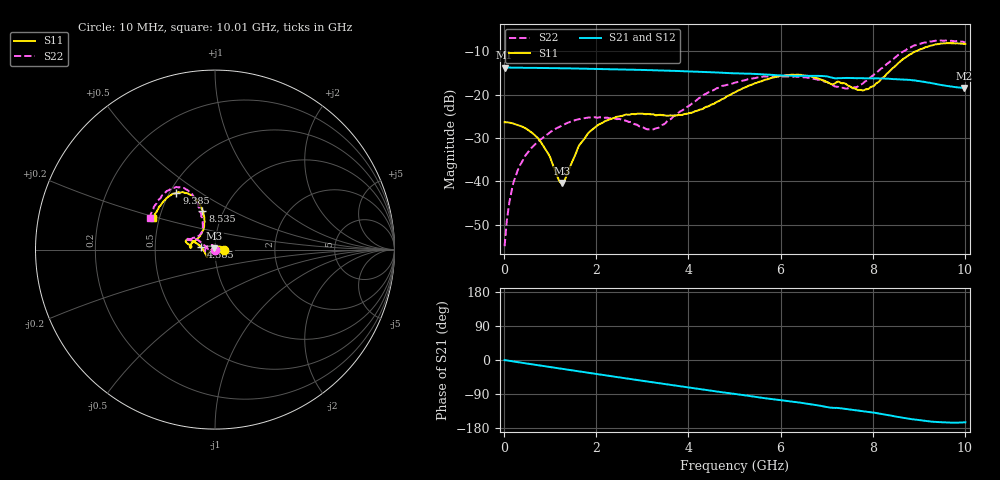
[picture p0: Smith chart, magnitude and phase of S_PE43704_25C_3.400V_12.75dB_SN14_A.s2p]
! Device ID: PE43704
! Dir: z:\PE43704\PE43704_Char_1_20130516\PE43704\AMB\3p400V\12p75dB
! Serial: 14
! Insertion: A
! Impedance: 50 ohm
! Temp: Amb
! VDD: 3.400V
! Attenuation Step: 12.75dB
! IDD: 1.140121e-01mA
#  Hz  S  RI  R  50
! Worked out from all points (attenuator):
!   401 points, 10 MHz to 10.01 GHz, reference 50 ohm
!   highest |S21| = -13.73 dB at 10 MHz (marker M1); lowest = -18.4 dB at 9.985 GHz (marker M2)
!   lowest |S11| = -40.4 dB at 1.26 GHz (marker M3), VSWR 1.02, Z = 49.5 + j0.822 ohm
!   |S11| at or under -10 dB: start of sweep to 8.933 GHz
!   |S22| runs from -54.9 to -7.5 dB; largest |S21 - S12| = 0.0015
!   S11 on the Smith chart (normalised r, x): 10 MHz: 1.10, +0.00; 4.585 GHz: 0.85, +0.03; 8.535 GHz: 0.80, +0.36; 9.385 GHz: 0.54, +0.40; 10.01 GHz: 0.46, +0.19
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1e7  0.0482 0.000196  0.2059 -0.000751  0.2061 -0.000737  0.00174 0.000404
1.6e8  0.0469 0.00473  0.2051 -0.0113  0.2052 -0.0111  0.00161 0.00748
3.6e8  0.0422 0.0106  0.2037 -0.0245  0.2035 -0.0247  -0.00204 0.0158
7.85e8  0.0233 0.0174  0.1969 -0.0516  0.1969 -0.0515  -0.0171 0.0251
1.26e9  -0.00475 0.0083  0.1854 -0.0803  0.1855 -0.0802  -0.0398 0.02
1.685e9  -0.0269 -0.00895  0.1715 -0.1037  0.1715 -0.1035  -0.0533 0.00488
2.01e9  -0.0375 -0.0222  0.1587 -0.1197  0.1588 -0.1196  -0.0541 -0.00553
2.41e9  -0.0427 -0.0344  0.141 -0.1373  0.141 -0.1372  -0.0516 -0.0116
3.135e9  -0.0456 -0.039  0.104 -0.1616  0.1041 -0.1616  -0.0398 -0.000886
3.36e9  -0.0475 -0.0344  0.0918 -0.1672  0.092 -0.1669  -0.0412 0.00657
3.885e9  -0.0571 -0.0148  0.0625 -0.1759  0.0627 -0.1758  -0.0618 0.0257
4.585e9  -0.0793 0.0156  0.023 -0.1793  0.0231 -0.1794  -0.1024 0.0561
5.01e9  -0.101 0.034  0.000993 -0.1765  0.00117 -0.1767  -0.1263 0.0549
5.96e9  -0.1533 0.0557  -0.0443 -0.1613  -0.0438 -0.1615  -0.1539 0.0525
6.685e9  -0.1573 0.0362  -0.0756 -0.1469  -0.0757 -0.1468  -0.1446 0.0529
7.56e9  -0.1078 0.0519  -0.1032 -0.1167  -0.1032 -0.1165  -0.0766 0.0914
7.885e9  -0.0769 0.0869  -0.1127 -0.1061  -0.1126 -0.1066  -0.0677 0.1315
8.36e9  -0.0598 0.1753  -0.1265 -0.0853  -0.1263 -0.086  -0.0842 0.2222
8.535e9  -0.0698 0.2172  -0.1302 -0.0759  -0.1297 -0.0766  -0.1025 0.2639
9.385e9  -0.2147 0.3164  -0.1271 -0.0377  -0.1274 -0.0369  -0.2515 0.3345
9.985e9  -0.3382 0.1847  -0.1155 -0.0318  -0.1163 -0.0316  -0.3592 0.1852
1.001e10  -0.3439 0.1746  -0.1162 -0.0322  -0.1168 -0.0322  -0.3629 0.1772
